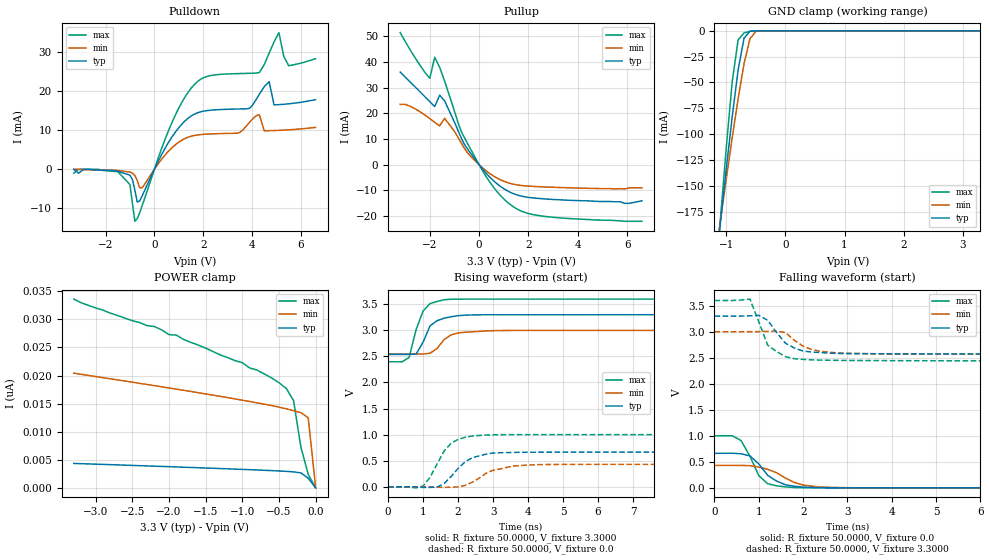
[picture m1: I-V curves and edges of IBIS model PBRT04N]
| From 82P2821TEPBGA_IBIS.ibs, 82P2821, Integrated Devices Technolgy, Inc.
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|   Model PBRT04N
[Model]		PBRT04N
Model_type	I/O
Polarity   Non-Inverting
Enable   Active-Low
Vinl = 		0.8000V
Vinh = 		2.0000V
C_comp   5.7300pF   5.2300pF   6.6100pF
[Temperature Range]	  25.0000   90.0000   -40.0000
[Voltage Range]   3.3000V   3.0000V   3.6000V
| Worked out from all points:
|   slope of the pulldown table from 0 to 0.495 V, typ, clamps not added: 82.7 ohm
|   slope of the pullup table from 0 to 0.495 V, typ, clamps not added: 91.5 ohm
|   GND clamp passes 1 mA (typ) near -0.61 V on its own axis
|   rising waveform, R_fixture 50.0000, V_fixture 3.3000: 20-80 % time 396ps typ, 428ps min, 333ps max; typ from 2.54 V to 3.3 V
|   rising waveform, R_fixture 50.0000, V_fixture 0.0: 20-80 % time 633ps typ, 820ps min, 540ps max; typ from 0 V to 0.664 V
|   falling waveform, R_fixture 50.0000, V_fixture 0.0: 20-80 % time 487ps typ, 636ps min, 372ps max; typ from 0.664 V to 0 V
|   falling waveform, R_fixture 50.0000, V_fixture 3.3000: 20-80 % time 485ps typ, 519ps min, 400ps max; typ from 3.3 V to 2.57 V
[Pulldown]
|Voltage	  I(typ)   I(min)   I(max)
-3.3V     0A         0A         -1mA
-1.5V     -500uA     -300uA     -600uA
-1V       -1.5mA     -700uA     -3.9mA
-800mV    -5.28mA    -1.58mA    -13.28mA
-500mV    -6.772mA   -4.745mA   -9.284mA
700mV     8.065mA    5.38mA     11.66mA
1.7V      14.26mA    8.709mA    22.03mA
4.3V      19.2mA     13.9mA     24.71mA
4.7V      22.37mA    9.863mA    29.69mA
5.1V      16.51mA    9.953mA    34.92mA
5.5V      16.73mA    10.09mA    26.45mA
6.6V      17.78mA    10.7mA     28.24mA
[Pullup]
|Voltage	  I(typ)   I(min)   I(max)
-3.2V     36.03mA    23.51mA    51.42mA
-2V       24.54mA    17.97mA    33.63mA
-1.8V     22.64mA    16.51mA    41.83mA
-1.6V     27.05mA    15.1mA     37.9mA
-1.4V     24.85mA    18.06mA    32.59mA
-700mV    9.882mA    8.072mA    12.47mA
-400mV    5.196mA    3.842mA    7.041mA
400mV     -4.493mA   -3.199mA   -6.275mA
1.2V      -10.42mA   -7.106mA   -15.02mA
1.8V      -12.37mA   -8.151mA   -18.37mA
2.6V      -13.26mA   -8.62mA    -20.02mA
6.6V      -14mA      -9mA       -22mA
[GND_clamp]
|Voltage	  I(typ)   I(min)   I(max)
-3.3V     -1.417A    -1.129A    -1.858A
-1.2V     -239.2mA   -225mA     -255.1mA
-1.1V     -185.7mA   -183.7mA   -182.6mA
-1V       -133.3mA   -143.1mA   -112.7mA
-900mV    -83.08mA   -103.5mA   -49.11mA
-800mV    -37.77mA   -65.73mA   -8.672mA
-700mV    -7.078mA   -31.8mA    -2.029mA
-600mV    -432.9uA   -7.712mA   -441uA
-500mV    -28.09uA   -557.2uA   -48.67uA
3.3V      948fA      13.74nA    -711.9pA
[POWER_clamp]
|Voltage	  I(typ)   I(min)   I(max)
-3.3V     4.351nA    20.42nA    33.61nA
-2.5V     4nA        18.82nA    29.76nA
-2.2V     3.863nA    18.2nA     28.73nA
-2V       3.773nA    17.79nA    27.29nA
-1.9V     3.725nA    17.58nA    27.21nA
-1V       3.292nA    15.61nA    22.3nA
-600mV    3.074nA    14.65nA    19.58nA
-400mV    2.937nA    14.08nA    17.72nA
-300mV    2.844nA    13.74nA    15.53nA
-200mV    2.662nA    13.39nA    7.239nA
-100mV    1.73nA     12.47nA    2.405nA
0V        951.1fA    202.7pA    683.6fA
[Ramp]
| variable   typ   min   max
dV/dt_r		0.3985/0.5965n   0.2582/0.8200n   0.6000/0.4893n
dV/dt_f		0.4392/0.4441n   0.2598/0.5043n   0.6984/0.3385n
R_load =	50.0000
[Rising Waveform]
R_fixture=	50.0000
V_fixture=	3.3000
V_fixture_min=	3.0000
V_fixture_max=	3.6000
|time   V(typ)   V(min)   V(max)
0s        2.539V     2.545V     2.398V
400ps     2.539V     2.545V     2.397V
600ps     2.539V     2.545V     2.48V
800ps     2.545V     2.545V     3.012V
1ns       2.774V     2.546V     3.372V
1.2ns     3.086V     2.562V     3.513V
1.6ns     3.233V     2.822V     3.587V
2ns       3.281V     2.951V     3.599V
3ns       3.3V       2.994V     3.599V
10ns      3.3V       3V         3.599V
[Rising Waveform]
R_fixture=	50.0000
V_fixture=	0.0
V_fixture_min=	0.0
V_fixture_max=	0.0
|time   V(typ)   V(min)   V(max)
0s        0V         0V         0V
1ns       -12.79mV   -498.8uV   13.86mV
1.2ns     -12.63mV   -3.104mV   182mV
1.4ns     -6.448mV   -7.79mV    437.3mV
1.6ns     62.56mV    -11.72mV   685.3mV
1.8ns     196.6mV    -9.397mV   834.5mV
2.4ns     555.5mV    85.97mV    973mV
3ns       647.5mV    316.8mV    997.7mV
3.6ns     658.8mV    399.5mV    1V
10ns      664.1mV    430.3mV    1V
[Falling Waveform]
R_fixture=	50.0000
V_fixture=	0.0
V_fixture_min=	0.0
V_fixture_max=	0.0
|time   V(typ)   V(min)   V(max)
0s        664.1mV    430.4mV    1V
400ps     665mV      430.5mV    1.001V
600ps     655.5mV    430.9mV    908.8mV
800ps     614.2mV    425.9mV    605.8mV
1ns       459.6mV    400.3mV    234.3mV
1.2ns     240.4mV    356mV      78.91mV
1.6ns     59.44mV    189.2mV    18.93mV
2ns       13.77mV    53.84mV    3.309mV
2.6ns     2.004mV    10.07mV    -90.25uV
10ns      -3.507uV   -952.7nV   -3.816uV
[Falling Waveform]
R_fixture=	50.0000
V_fixture=	3.3000
V_fixture_min=	3.0000
V_fixture_max=	3.6000
|time   V(typ)   V(min)   V(max)
0s        3.3V       3V         3.6V
800ps     3.305V     3.001V     3.626V
1ns       3.314V     3.002V     3.19V
1.2ns     3.219V     3.007V     2.741V
1.6ns     2.78V      2.983V     2.521V
1.8ns     2.688V     2.837V     2.481V
2ns       2.628V     2.72V      2.467V
2.2ns     2.609V     2.656V     2.458V
2.8ns     2.582V     2.59V      2.449V
10ns      2.568V     2.567V     2.436V
